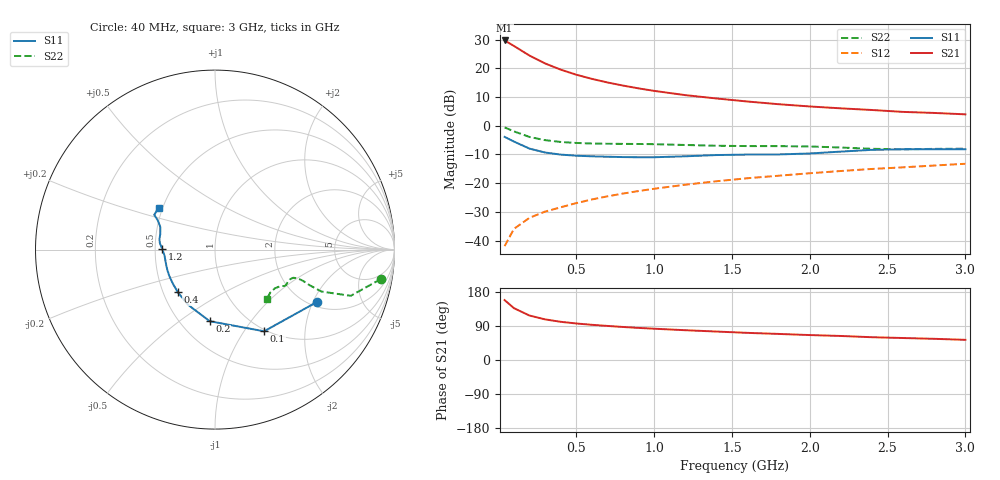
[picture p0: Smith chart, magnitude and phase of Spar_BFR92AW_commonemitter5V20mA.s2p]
! Filename:  BFR92AWE.S2P  Version:  4.0
! NXP part #: BFR92AW  Date: Jun 1994
! Bias condition: Vce=5V, Ic=20mA
#  MHz  S  MA  R  50
! Freq  S11  S21  S12  S22  !GUM [dB]
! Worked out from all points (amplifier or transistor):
!   21 points, 40 MHz to 3 GHz, reference 50 ohm
!   highest |S21| = 29.7 dB at 40 MHz (marker M1)
!   |S21| within 3 dB of that: start of sweep to 132.2 MHz
!   unconditionally stable (mu >= 1): 461.3 MHz to end of sweep
!   at 300 MHz: K = 0.85, MSG = 25.8 dB, |S12| = -29.9 dB
!   at 1 GHz: K = 1.12, MAG = 14.9 dB, |S12| = -21.9 dB
!   at 3 GHz: K = 1.07, MAG = 7.0 dB, |S12| = -13.2 dB
!   S11 on the Smith chart (normalised r, x): 40 MHz: 2.19, -2.16; 100 MHz: 0.98, -1.24; 200 MHz: 0.69, -0.65; 400 MHz: 0.59, -0.31; 1.2 GHz: 0.55, +0.01; 3 GHz: 0.48, +0.26
40  0.64 -27.0  30.62 158.1  0.008 79.1  0.938 -10.1
100  0.531 -59.0  24.55 136.8  0.016 67.8  0.799 -18.8
200  0.4 -94.2  16.7 117.3  0.025 63.6  0.638 -21.5
300  0.342 -116.1  12.19 107.2  0.032 64.4  0.562 -20.6
400  0.315 -131.4  9.503 100.8  0.038 66.9  0.523 -19.6
500  0.301 -141.7  7.76 96.4  0.045 68.5  0.502 -19.3
600  0.294 -150.1  6.567 92.9  0.052 70.7  0.491 -19.3
700  0.289 -156.5  5.688 89.9  0.059 71.9  0.486 -19.4
800  0.285 -162.5  5.019 87.2  0.066 73.1  0.484 -19.5
900  0.283 -168.0  4.485 84.7  0.073 73.7  0.482 -19.4
1000  0.283 -172.8  4.054 82.6  0.08 74.4  0.478 -19.4
1200  0.294 179.1  3.42 78.6  0.094 75.1  0.463 -19.8
1400  0.309 173.5  2.991 75.1  0.108 75.9  0.449 -21.7
1600  0.315 169.2  2.647 71.6  0.122 76.0  0.443 -24.8
1800  0.317 164.1  2.375 68.8  0.135 76.5  0.442 -26.7
2000  0.329 157.7  2.17 65.8  0.149 76.7  0.436 -27.7
2200  0.355 153.3  2.012 63.4  0.163 77.0  0.418 -29.1
2400  0.381 150.9  1.883 60.1  0.177 77.2  0.397 -32.9
2600  0.39 150.3  1.745 58.0  0.189 76.8  0.39 -38.1
2800  0.39 148.0  1.673 55.9  0.203 77.4  0.396 -41.8
3000  0.39 143.5  1.582 53.2  0.218 77.5  0.399 -44.0
